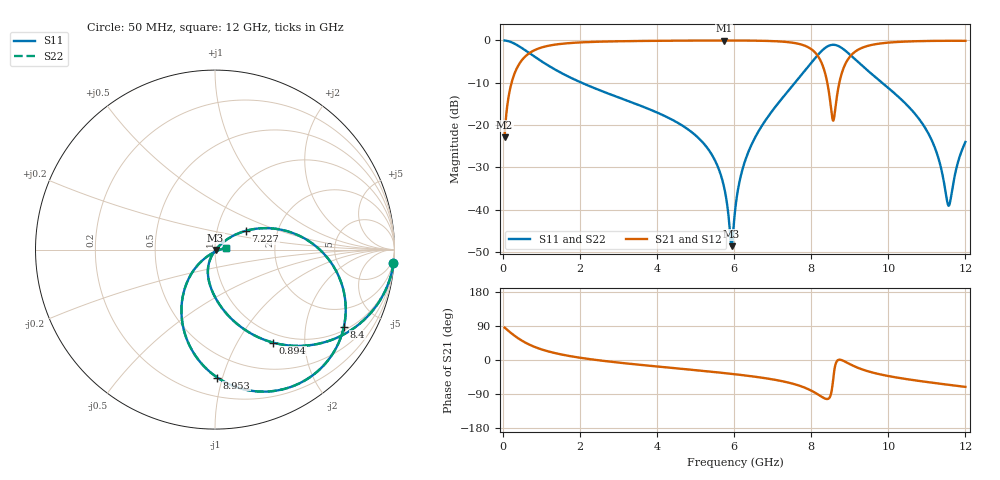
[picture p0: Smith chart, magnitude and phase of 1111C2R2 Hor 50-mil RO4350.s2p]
# GHz S MA R 50
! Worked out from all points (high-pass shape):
!   1601 points, 50 MHz to 12 GHz, reference 50 ohm
!   highest |S21| = -0.03 dB at 5.741 GHz (marker M1); lowest = -22.9 dB at 50 MHz (marker M2)
!   |S21| within 3 dB of the highest: 689.7 MHz to 8.118 GHz (7.428 GHz wide, 169 % of centre); 9.091 GHz to end of sweep
!   lowest |S11| = -48.6 dB at 5.935 GHz (marker M3), VSWR 1.01, Z = 50.3 - j0.236 ohm
!   |S11| at or under -10 dB: 2.045 GHz to 7.581 GHz (5.537 GHz wide, 115 % of centre); 9.838 GHz to end of sweep
!   |S22| runs from -48.6 to 0.0 dB; largest |S21 - S12| = 0
!   S11 on the Smith chart (normalised r, x): 50 MHz: 1, -26; 894 MHz: 0.86, -1.43; 7.227 GHz: 1.38, +0.30; 8.4 GHz: 1.14, -3.26; 8.953 GHz: 0.33, -0.96; 12 GHz: 1.13, +0.02
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0.05  0.9974 -4.4  0.07196 85.5  0.07196 85.5  0.9974 -4.4
0.1769688  0.9688 -15.5  0.2474 74.5  0.2474 74.5  0.9688 -15.5
0.3263437  0.9045 -27.3  0.426 62.7  0.426 62.7  0.9045 -27.3
0.8939687  0.6117 -57.9  0.7901 32.0  0.7901 32.0  0.6117 -57.9
2.044156  0.3163 -84.4  0.9472 5.4  0.9472 5.4  0.3163 -84.4
4.038312  0.1383 -106.6  0.9882 -17.5  0.9882 -17.5  0.1383 -106.6
5.203437  0.06126 -116.3  0.9951 -28.9  0.9951 -28.9  0.06126 -116.3
5.741187  0.01851 -114.0  0.9961 -34.5  0.9961 -34.5  0.01851 -114.0
5.935375  0.003707 -39.4  0.996 -36.6  0.996 -36.6  0.003707 -39.4
6.025  0.009566 28.4  0.9957 -37.6  0.9957 -37.6  0.009566 28.4
6.159438  0.02334 40.4  0.9952 -39.2  0.9952 -39.2  0.02334 40.4
6.3835  0.04955 42.4  0.9936 -42.0  0.9936 -42.0  0.04955 42.4
7.227469  0.2016 31.3  0.9678 -55.5  0.9678 -55.5  0.2016 31.3
8.019156  0.5548 2.6  0.7775 -81.6  0.7775 -81.6  0.5548 2.6
8.400063  0.8365 -30.8  0.3472 -102.9  0.3472 -102.9  0.8365 -30.8
8.579313  0.8869 -52.0  0.1136 -43.8  0.1136 -43.8  0.8869 -52.0
8.95275  0.7129 -89.0  0.5953 -8.2  0.5953 -8.2  0.7129 -89.0
9.333656  0.4969 -109.8  0.8214 -25.2  0.8214 -25.2  0.4969 -109.8
10.01331  0.271 -128.1  0.9414 -42.5  0.9414 -42.5  0.271 -128.1
11.05894  0.07653 -139.5  0.9842 -58.8  0.9842 -58.8  0.07653 -139.5
11.55934  0.01118 -70.1  0.9883 -65.4  0.9883 -65.4  0.01118 -70.1
12  0.063 9.4  0.987 -71.0  0.987 -71.0  0.063 9.4
